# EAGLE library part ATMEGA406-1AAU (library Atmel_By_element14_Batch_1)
8-bit Microcontroller with 40K Bytes In-System Programmable Flash
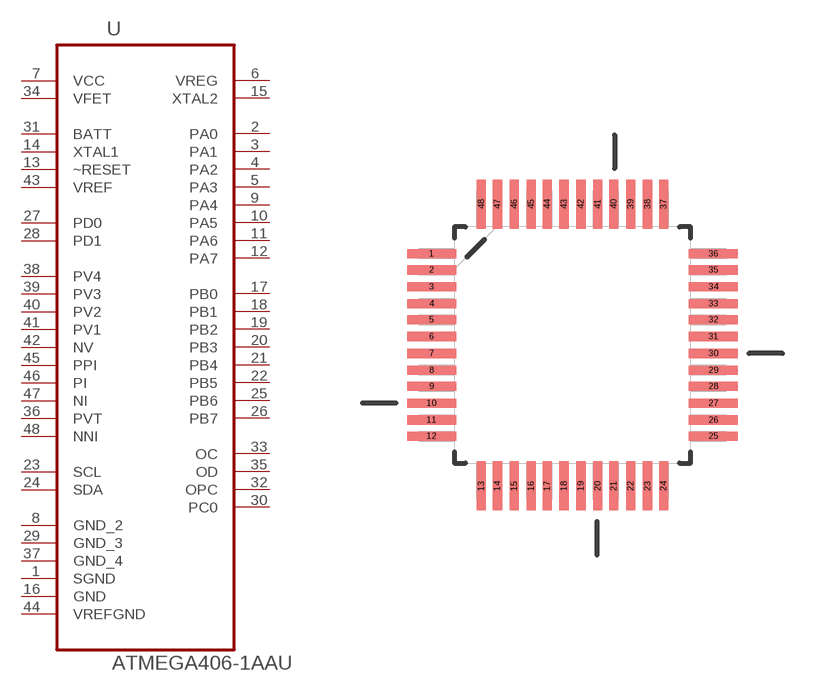
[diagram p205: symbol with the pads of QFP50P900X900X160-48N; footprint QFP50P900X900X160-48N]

Designator prefix U

## ATMEGA406-1AAU (MPN: ATMEGA406-1AAU; OC_FARNELL: 1455115; OC_NEWARK: 58M3739; PACKAGE: LQFP-48; SUPPLIER: Atmel)  [QFP50P900X900X160-48N]
1  SGND  pas
2  PA0
3  PA1
4  PA2
5  PA3
6  VREG
7  VCC  pwr
8  GND_2  pas
9  PA4
10  PA5
11  PA6
12  PA7
13  ~RESET  in
14  XTAL1  in
15  XTAL2  out
16  GND  pas
17  PB0
18  PB1
19  PB2
20  PB3
21  PB4
22  PB5
23  SCL
24  SDA
25  PB6
26  PB7
27  PD0
28  PD1
29  GND_3  pas
30  PC0
31  BATT  in
32  OPC  out
33  OC  out
34  VFET  pwr
35  OD  out
36  PVT  in
37  GND_4  pas
38  PV4  in
39  PV3  in
40  PV2  in
41  PV1  in
42  NV  in
43  VREF  pwr
44  VREFGND  pas
45  PPI  in
46  PI  in
47  NI  in
48  NNI  in

## Footprint QFP50P900X900X160-48N (pad centres in mm)
smd 1.473 x 0.279: 1 -4.242,2.743; 2 -4.242,2.261; 3 -4.242,1.753; 4 -4.242,1.245; 5 -4.242,0.762; 6 -4.242,0.254; 7 -4.242,-0.254; 8 -4.242,-0.762; 9 -4.242,-1.245; 10 -4.242,-1.753; 11 -4.242,-2.261; 12 -4.242,-2.743; 25 4.242,-2.743; 26 4.242,-2.261; 27 4.242,-1.753; 28 4.242,-1.245; 29 4.242,-0.762; 30 4.242,-0.254; 31 4.242,0.254; 32 4.242,0.762; 33 4.242,1.245; 34 4.242,1.753; 35 4.242,2.261; 36 4.242,2.743
smd 0.279 x 1.473: 13 -2.743,-4.242; 14 -2.261,-4.242; 15 -1.753,-4.242; 16 -1.245,-4.242; 17 -0.762,-4.242; 18 -0.254,-4.242; 19 0.254,-4.242; 20 0.762,-4.242; 21 1.245,-4.242; 22 1.753,-4.242; 23 2.261,-4.242; 24 2.743,-4.242; 37 2.743,4.242; 38 2.261,4.242; 39 1.753,4.242; 40 1.245,4.242; 41 0.762,4.242; 42 0.254,4.242; 43 -0.254,4.242; 44 -0.762,4.242; 45 -1.245,4.242; 46 -1.753,4.242; 47 -2.261,4.242; 48 -2.743,4.242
